FUNCTION_BLOCK "Add_Int"
VERSION : 0.1
   VAR_INPUT
      "I0.0" : Int;
      "I0.1" : Int;
   END_VAR

   VAR_OUTPUT
      "O0.0" : Int;
   END_VAR


BEGIN
NETWORK
TITLE =
      L #"I0.0";
      L #"I0.1";
      +I;
      T #"O0.0";
      NOP 0;
NETWORK
TITLE =
END_FUNCTION_BLOCK

